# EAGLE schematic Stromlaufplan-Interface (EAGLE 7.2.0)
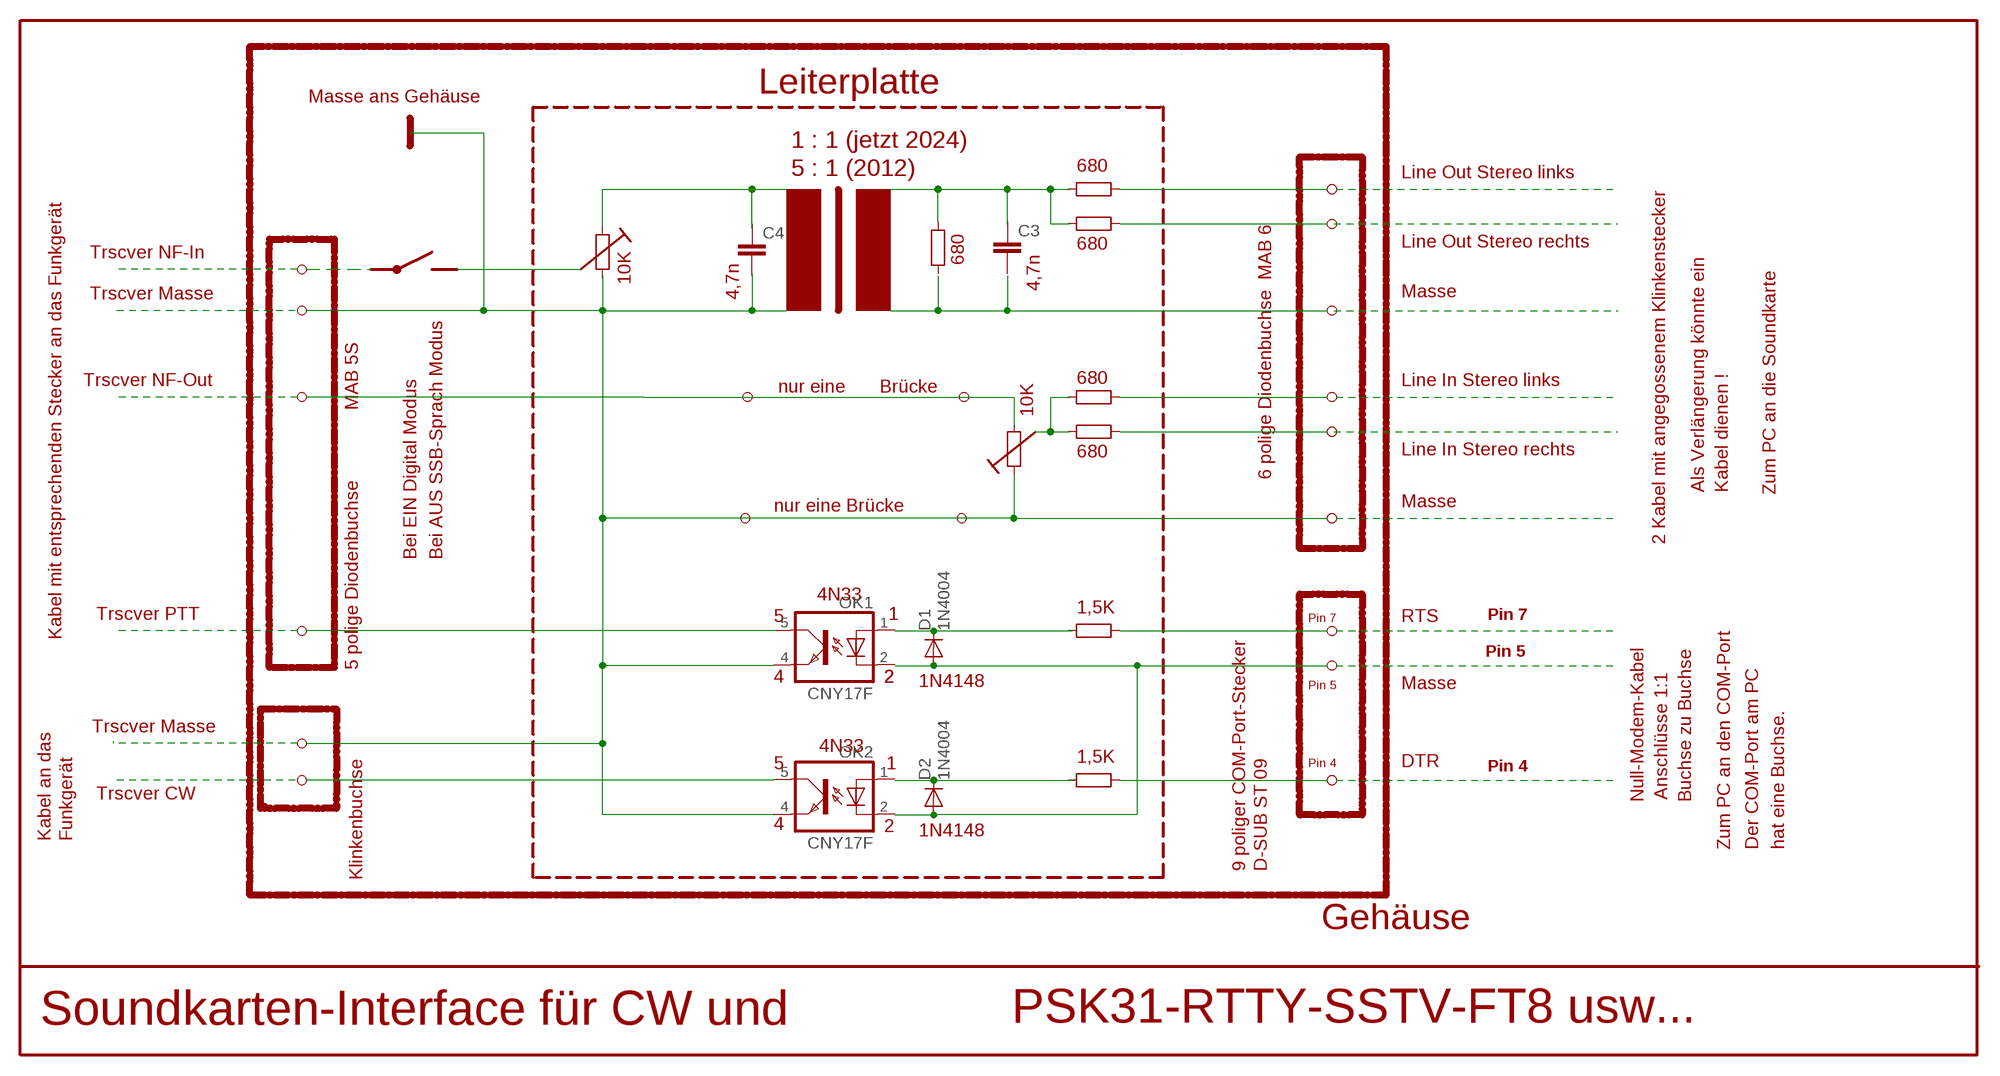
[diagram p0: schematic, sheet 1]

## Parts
C3  C2,5-3  [C2.5-3]
C4  C2,5-3  [C2.5-3]
D1  1N4004  [DO41-10]
D2  1N4004  [DO41-10]
OK1  CNY17F  [DIL06]
OK2  CNY17F  [DIL06]

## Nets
N$1: C3.1
N$2: D1.C
N$4: D1.A D2.A
N$13: C4.1
N$16: OK2.5(COL)
N$17: D2.C
N$18: C4.2
N$38: OK1.5(COL)
Unconnected: C3.2 OK1.1(A) OK1.2(C) OK1.4(EMIT) OK2.1(A) OK2.2(C) OK2.4(EMIT)

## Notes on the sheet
- Leiterplatte
- Masse ans Gehäuse
- 1 : 1 (jetzt 2024)
- 5 : 1 (2012) | 680
- Line Out Stereo links
- 680 | Line Out Stereo rechts
- Trscver NF-In
- 680
- 10K
- 4,7n
- Trscver Masse | 4,7n | Masse
- Trscver NF-Out | 680 | Line In Stereo links
- nur eine | Brücke
- MAB 5S
- 10K
- 680 | Line In Stereo rechts
- 6 polige Diodenbuchse  MAB 6
- Als Verlängerung könnte ein | Kabel dienen ! | Zum PC an die Soundkarte
- nur eine Brücke | Masse
- 2 Kabel mit angegossenem Klinkenstecker
- Bei EIN Digital Modus | Bei AUS SSB-Sprach Modus
- 4N33
- 1,5K
- Trscver PTT | 5 | 1 | Pin 7 | RTS | Pin 7
- Kabel mit entsprechenden Stecker an das Funkgerät
- Pin 5
- 5 polige Diodenbuchse
- 4 | 2 | 2 | 1N4148
- Pin 5 | Masse
- Trscver Masse
- 4N33
- 1,5K
- 5 | 1 | Pin 4 | DTR
- Pin 4
- Trscver CW | Null-Modem-Kabel | Anschlüsse 1:1 | Buchse zu Buchse
- 4 | 2
- Kabel an das | Funkgerät | 1N4148
- Zum PC an den COM-Port | Der COM-Port am PC | hat eine Buchse.
- 9 poliger COM-Port-Stecker | D-SUB ST 09
- Klinkenbuchse
- Gehäuse
- Soundkarten-Interface für CW und | PSK31-RTTY-SSTV-FT8 usw...

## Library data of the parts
C3 C4 = capacitor-wima:C: CAPACITOR
D1 D2 = diode:1N4004: DIODE
OK1 OK2 = optocoupler:CNY17F: SIEMENS OPTO COUPLER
